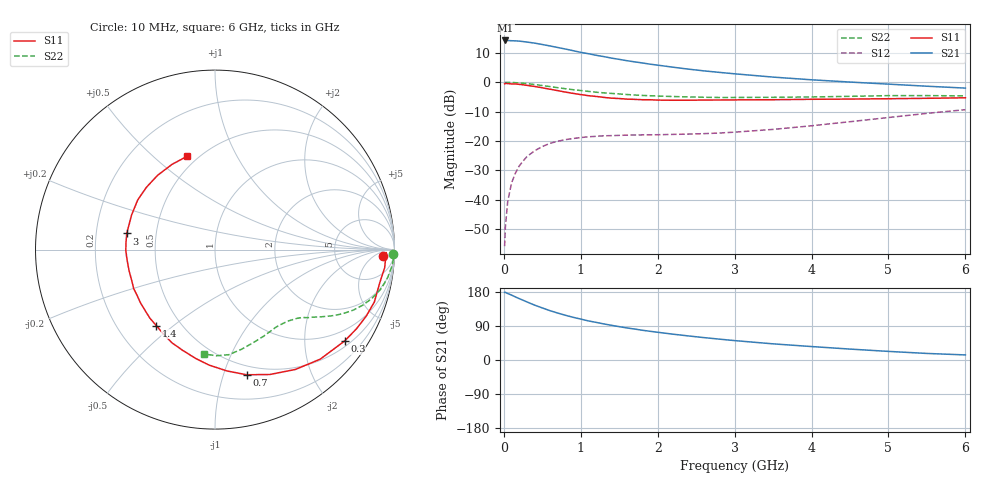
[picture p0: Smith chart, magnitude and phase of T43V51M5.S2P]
! Infineon Technologies  Discrete & RF Semiconductors
! BFR182T
! Si NPN RF Bipolar Junction Transistor in SC75
! VCE = 3.5 V  IC = 1.5 mA
! Common Emitter S-Parameters:  October  1999
# GHz  S  MA  R  50
!  f  S11  S21  S12  S22
! GHz  MAG  ANG  MAG  ANG  MAG  ANG  MAG  ANG
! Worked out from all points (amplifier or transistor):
!   36 points, 10 MHz to 6 GHz, reference 50 ohm
!   highest |S21| = 14.2 dB at 20 MHz (marker M1)
!   |S21| within 3 dB of that: start of sweep to 813.5 MHz
!   unconditionally stable (mu >= 1): 2.173 GHz to 4.436 GHz
!   at 250 MHz: K = 0.12, MSG = 20.4 dB, |S12| = -26.9 dB
!   at 1.4 GHz: K = 0.69, MSG = 13.2 dB, |S12| = -18.2 dB
!   at 6 GHz: K = 0.83, MSG = 3.7 dB, |S12| = -9.4 dB
!   S11 on the Smith chart (normalised r, x): 10 MHz: 23, -14; 300 MHz: 0.65, -3.03; 700 MHz: 0.41, -1.20; 1.4 GHz: 0.37, -0.44; 3 GHz: 0.34, +0.08; 6 GHz: 0.44, +0.65
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0.01  0.9393 -2.2  5.116 178.5  0.0016 79.2  0.9911 -1.3
0.02  0.9545 -1.0  5.157 178.6  0.0034 100.5  0.9904 -0.8
0.05  0.9506 -6.1  5.145 175.5  0.0092 89.2  0.9957 -2.5
0.1  0.9359 -11.6  5.102 171.3  0.0191 83.4  0.9922 -4.8
0.2  0.9206 -23.7  5.026 162.0  0.0373 77.4  0.9735 -9.4
0.3  0.884 -35.1  4.84 153.3  0.0539 70.8  0.9479 -13.6
0.4  0.8462 -46.2  4.647 144.8  0.0678 64.3  0.9137 -17.5
0.5  0.8038 -56.2  4.399 137.4  0.08 59.3  0.8783 -20.7
0.6  0.7599 -66.3  4.158 130.2  0.0907 55.3  0.8429 -23.5
0.7  0.7193 -75.8  3.913 123.9  0.0986 51.4  0.807 -25.9
0.9  0.6447 -92.8  3.452 112.7  0.1096 45.1  0.7457 -29.7
1.1  0.5895 -107.8  3.062 103.1  0.1175 41.1  0.6977 -32.5
1.4  0.5351 -127.6  2.579 91.5  0.1228 37.2  0.6445 -36.0
1.6  0.5152 -139.7  2.328 84.6  0.1252 36.1  0.617 -37.8
1.8  0.503 -150.1  2.133 78.5  0.1265 36.3  0.5952 -40.1
2.2  0.4929 -166.2  1.804 68.1  0.1289 38.1  0.5704 -44.2
2.6  0.4969 -179.5  1.563 59.1  0.1328 41.7  0.5544 -49.2
3  0.4997 169.6  1.392 51.2  0.1408 46.3  0.5496 -53.9
3.5  0.5032 157.5  1.223 42.6  0.1568 52.1  0.5534 -60.8
4.5  0.5163 137.8  1.007 28.8  0.2122 58.8  0.5746 -75.1
5.5  0.5319 116.7  0.855 17.3  0.2945 58.2  0.5915 -89.3
6  0.5428 106.5  0.794 13.4  0.3404 55.5  0.5847 -95.9
